(* Logix 5000 AddOnInstructionDefinition export Banner_QCM50_Param_v4; software revision 33.00 *)

TYPE Banner_IOL_Port_v4 :   // UDT that has all of the data items necessary to communicate with a specific Port on a IO-Link Master
STRUCT
   Port_Controlled : INT;   // Each bit represents a port on an IO-Link Master. Set to 1 to tell AOI to control that port.
   Port_Activate : INT;   // Each bit represents a port on an IO-Link Master. When ON that port will process any commands in queue.
   Port_Read : INT;   // Each bit represents a port on an IO-Link Master. Used to determine when device AOI has requested a Read command.
   Port_Write : INT;   // Each bit represents a port on an IO-Link Master. Used to determine when device AOI has requested a Write command.
   Port_RW_Complete : INT;   // Each bit represents a port on an IO-Link Master. Tells device AOI that Read or Write request has been completed.
   Port_Device_Read : INT;
   Data_Transfer : SINT[190];   // Array to transfer data from IO-Master to device AOIs.
END_STRUCT
END_TYPE

TYPE Banner_QCM50_Color_Tol_v4 :   // Color Tolerances for a QCM50.
STRUCT
   Ratio_Red : INT;   // 0 to 4095 = 0 to 100%
   Ratio_Green : INT;   // 0 to 4095 = 0 to 100%
   Energy : INT;   // 0 to 4095 = 0 to 100%
   Red_Tolerance : INT;   // 0 to 4095 = 0 to 100%
   Green_Tolerance : INT;   // 0 to 4095 = 0 to 100%
   Energy_Tolerance : INT;   // 0 to 4095 = 0 to 100%
END_STRUCT
END_TYPE

TYPE Banner_QCM50_Color_v4 :
STRUCT
   Tolerance : INT;   // 0 = Finest, 1 = 2nd level, 2 = 3rd level, 3 = 4th level, 4 = 5th level, 5 = 6th level, 6 = 7th level, 7 = 8th level, 8 = Roughest level
   NO_NC : SINT;   // 0 = NO, 1 = NC
   Function_Switching_Output : SINT;   // 0 = Disable, 1 = Output
   Energy_Evalution : SINT;   // 0 = Off, 1 = On
   Counter : DINT;   // 0 to 65535
   On_Delay : DINT;   // 0 to 65535
   Off_Delay : DINT;   // 0 to 65535
   Impulse_1Shot : DINT;   // 0 to 65535
   Connect_Colors : SINT;   // See IODD for more information.
END_STRUCT
END_TYPE

TYPE Banner_QCM50_RD_v4 :   // UDT that stores the Write Data for a QCM50.
STRUCT
   Master_Cycle_Time : INT;
   Min_Cycle_Time : INT;
   M_Sequence_Capability : INT;
   IO_Link_Version_ID : INT;
   Process_Data_Input_Length : INT;
   Process_Data_Output_Length : INT;
   Combined_Vendor_ID : DINT;   // IO-Link Vendor ID
   Vendor_ID1 : INT;
   Vendor_ID2 : INT;
   Combined_Device_ID : DINT;   // IO-Link Device ID
   Device_ID1 : INT;
   Device_ID2 : INT;
   Device_ID3 : INT;
   Serial_Number : STRING;
   Operating_Temp : INT;
   Max_Temp_Since_Restart : INT;
   Min_Temp_Since_Restart : INT;
   Max_Temp_Lifetime : INT;
   Min_Temp_Lifetime : INT;
   Operating_Hours : DINT;
   Counter_Switch_Cycle : DINT;
   Teach_Status : SINT;   // 0 = Idle, 1 to 3 = Success, 4 = Wait for Command, 5 = Busy, 7 = Error
   SP1_TP1 : SINT;   // 0 = -, 1 = Teach Successful.
   SP1_TP2 : SINT;   // 0 = -, 1 = Teach Successful.
   SP2_TP1 : SINT;   // 0 = -, 1 = Teach Successful.
   SP2_TP2 : SINT;   // 0 = -, 1 = Teach Successful.
   Current_Signal_Quality : INT;   // 0 to 100
END_STRUCT
END_TYPE

TYPE Banner_QCM50_v4 :   // All of the parameters for a QCM50.
STRUCT
   Initial_Global_Read : BOOL;   // Determines if all of the IO-Link data has been read into the PLC yet
   Command : INT;   // Value placed in here will activate a read or write to a specifc IO-Link Index
   Read_Data : Banner_QCM50_RD_v4;   // Read Only Data
   Write_Data : Banner_QCM50_WD_v4;   // Write Data
   Archive : Banner_QCM50_WD_v4;   // Archive of Write Data. Used to determine when data needs to be updated in the IO-Link Master.
   Reset : BOOL;   // Resets AOI. This will force a complete parameter read of the sensor.
END_STRUCT
END_TYPE

TYPE Banner_QCM50_WD_v4 :   // UDT that stores the Write Data for a Q4X.
STRUCT
   System_Command : INT;   // See IODD file for list of commands that can be activated via the System Command interface
   Parameter_Access_Lock : SINT;   // Write access to all parameters is prohibited while value is 1. Only this parameter can be adjusted when value is 1.
   Data_Storage_Lock : SINT;   // Automatic data storage is disabled when this value is equal to 1. Read access is not affected.
   Local_Parameterization_Lock : SINT;   // Parameterization via local control elements on device is disabled.
   Local_User_Interface_Lock : SINT;   // Operation of local user interface is disabled.
   Color_Setpoint : Banner_QCM50_Color_v4[13];
   Color1_Tolerances : Banner_QCM50_Color_Tol_v4[13];
   PNP_NPN : SINT;   // 0 = NPN, 1 = PNP, 2 = Auto
   Switching_Freq_Averaging : SINT;   // 0 = 3 Hz, 1 = 30 Hz, 2 = 100 Hz, 3 = 300 Hz, 4 = 500 Hz, 5 = 1500 Hz, 6 = 3000 Hz
   Binary_Output : SINT;   // 0 = Disable, 1 = Enable. NA for K1.
   Detection_Mode : SINT;   // 0 = Color Mode, 1 = Best Fit. NA for K1.
   Signal_Quality_Level : SINT;   // 10 to 90
   Process_Data_Mapping : SINT;   // 0 = Switching Channel, 1 = Color Values. NA for K1.
   Teach_Channel : SINT;   // Check IODD files for options. NA for K1.
   Input_Config : SINT;   // 0 = Disable Input, 2 = Key Lock, 3 = Trigger, 4 = External Teach. NA for K2 and K3.
   Screensaver : SINT;   // 0 = Screensaver Off, 1 = Screensaver On
   Rotate_Display : SINT;   // 0 = Display read from back, 1 = Dispalay read from front
END_STRUCT
END_TYPE

ADD_ON_INSTRUCTION Banner_QCM50_Param_v4   (* revision 4.0, vendor Banner Engineering *)
// AOI to read and write parameter data to an IO-Link QCM50.
VAR_IN_OUT
   QCM50 : Banner_QCM50_v4; {required}
   Port_Data : Banner_IOL_Port_v4; {required}
END_VAR
VAR_INPUT
   Port : INT; {required}   // Enter the Port number that this AOI is to work with.
   K : SINT; {required}   // 1,3,or 5. Based off number after the K in part number.
END_VAR
VAR
   Local_Control : DINT; {access None}
   Global_Read_Command_Value : INT; {access None}
   Global_Write_Command_Value : INT; {access None}
   Command_Being_Processed : BOOL; {access None}
   Update_Archive : BOOL; {access None}
   Index_Write_Inprocess : DINT; {access None}
   Index_Write_Control : DINT; {access None}
   Inprocess_Index : DINT; {access None}
   CR_Index : SINT; {access None}
   CWC3_Index : SINT; {access None}
   CWC2_Index : SINT; {access None}
   CWC1_Index : SINT; {access None}
   C_Limit : SINT[2]; {access None}
   ColorChange : SINT[3] := ([0] := 1, [1] := 7, [2] := 12); {access None}
   CW_Index : SINT; {access None}
END_VAR

ROUTINE Logic   (* ladder *)
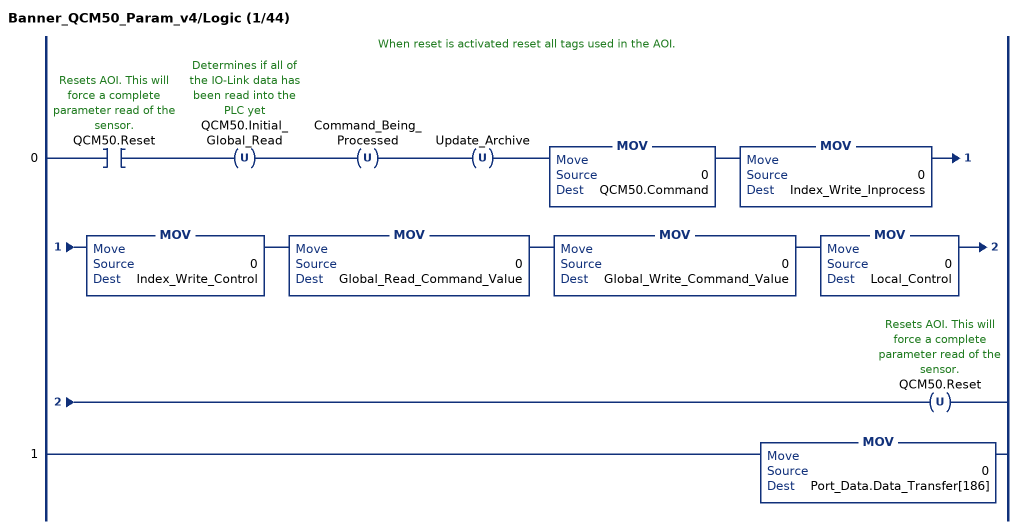
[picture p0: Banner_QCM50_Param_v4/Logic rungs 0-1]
   // When reset is activated reset all tags used in the AOI.
   0: XIC(QCM50.Reset)OTU(QCM50.Initial_Global_Read)OTU(Command_Being_Processed)OTU(Update_Archive)MOV(0,QCM50.Command)MOV(0,Index_Write_Inprocess)MOV(0,Index_Write_Control)MOV(0,Global_Read_Command_Value)MOV(0,Global_Write_Command_Value)MOV(0,Local_Control)OTU(QCM50.Reset);
   1: MOV(0,Port_Data.Data_Transfer[186]);
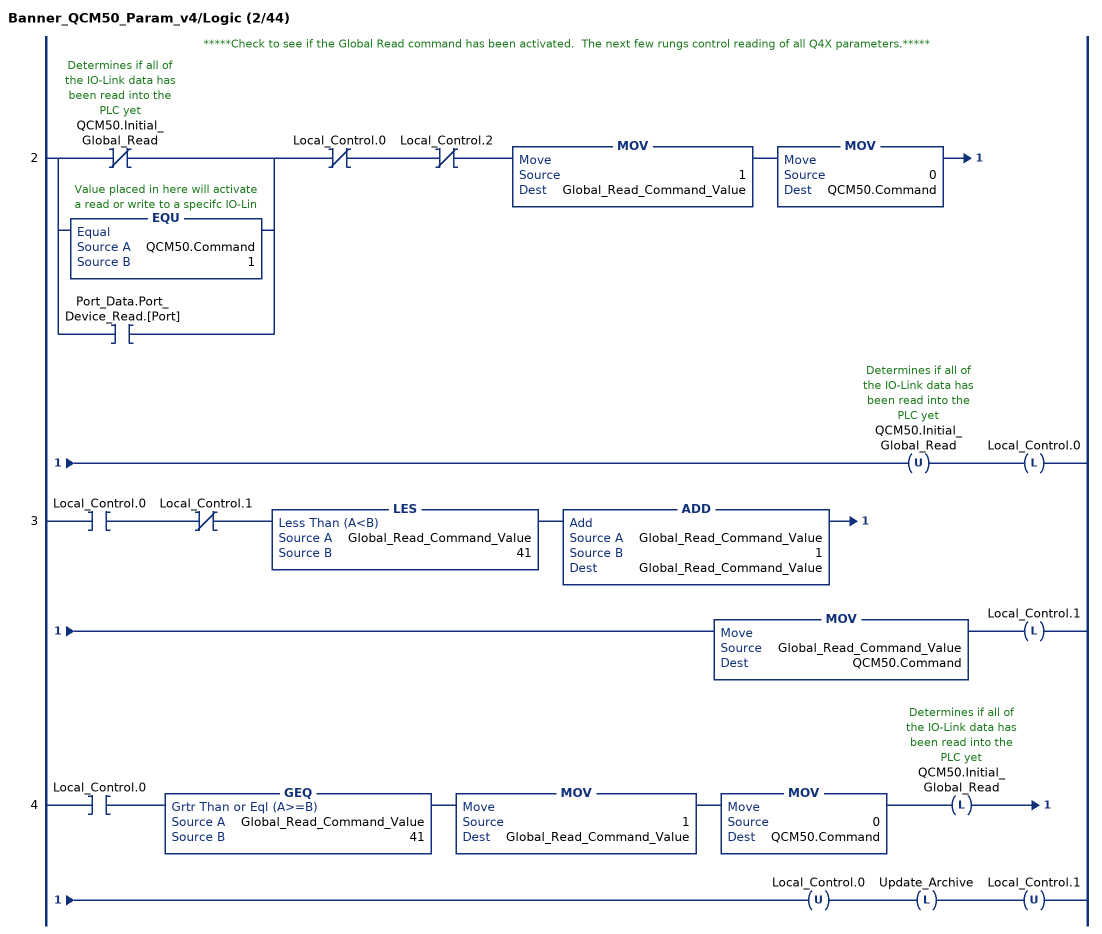
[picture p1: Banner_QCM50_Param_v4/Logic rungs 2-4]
   // *****Check to see if the Global Read command has been activated.  The next few rungs control reading of all Q4X parameters.*****
   2: [XIO(QCM50.Initial_Global_Read) ,EQU(QCM50.Command,1) ,XIC(Port_Data.Port_Device_Read.[Port]) ]XIO(Local_Control.0)XIO(Local_Control.2)MOV(1,Global_Read_Command_Value)MOV(0,QCM50.Command)OTU(QCM50.Initial_Global_Read)OTL(Local_Control.0);
   3: XIC(Local_Control.0)XIO(Local_Control.1)LES(Global_Read_Command_Value,41)ADD(Global_Read_Command_Value,1,Global_Read_Command_Value)MOV(Global_Read_Command_Value,QCM50.Command)OTL(Local_Control.1);
   4: XIC(Local_Control.0)GEQ(Global_Read_Command_Value,41)MOV(1,Global_Read_Command_Value)MOV(0,QCM50.Command)OTL(QCM50.Initial_Global_Read)OTU(Local_Control.0)OTL(Update_Archive)OTU(Local_Control.1);
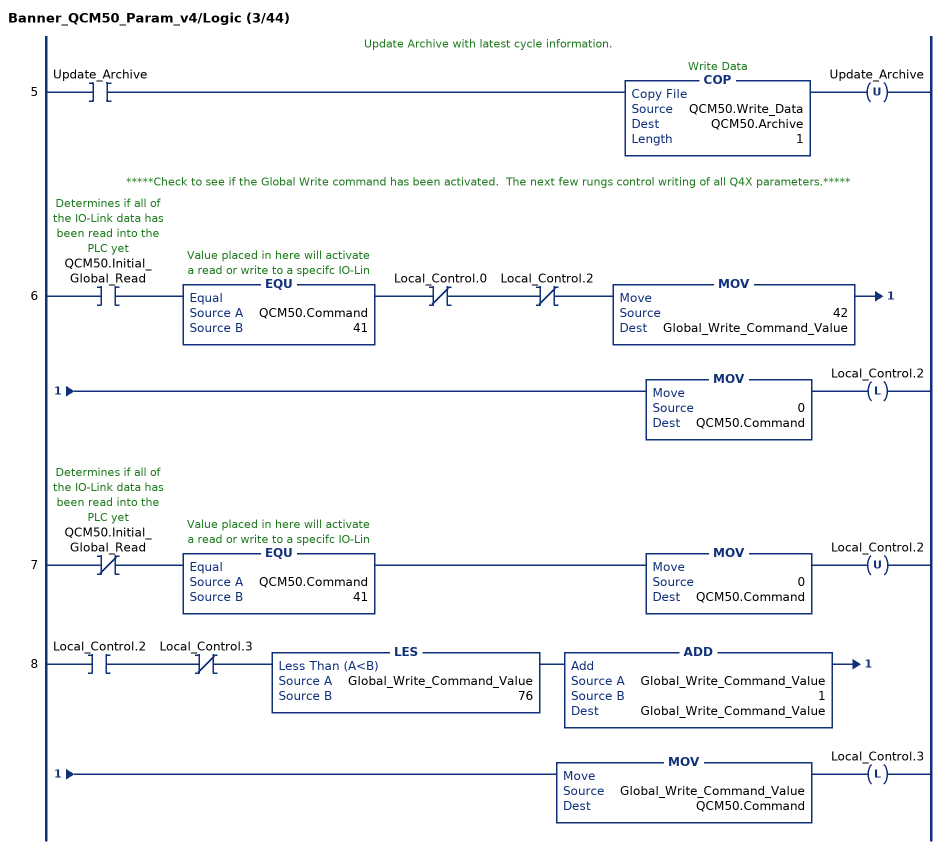
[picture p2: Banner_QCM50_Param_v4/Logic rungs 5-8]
   // Update Archive with latest cycle information.
   5: XIC(Update_Archive)COP(QCM50.Write_Data,QCM50.Archive,1)OTU(Update_Archive);
   // *****Check to see if the Global Write command has been activated.  The next few rungs control writing of all Q4X parameters.*****
   6: XIC(QCM50.Initial_Global_Read)EQU(QCM50.Command,41)XIO(Local_Control.0)XIO(Local_Control.2)MOV(42,Global_Write_Command_Value)MOV(0,QCM50.Command)OTL(Local_Control.2);
   7: XIO(QCM50.Initial_Global_Read)EQU(QCM50.Command,41)MOV(0,QCM50.Command)OTU(Local_Control.2);
   8: XIC(Local_Control.2)XIO(Local_Control.3)LES(Global_Write_Command_Value,76)ADD(Global_Write_Command_Value,1,Global_Write_Command_Value)MOV(Global_Write_Command_Value,QCM50.Command)OTL(Local_Control.3);
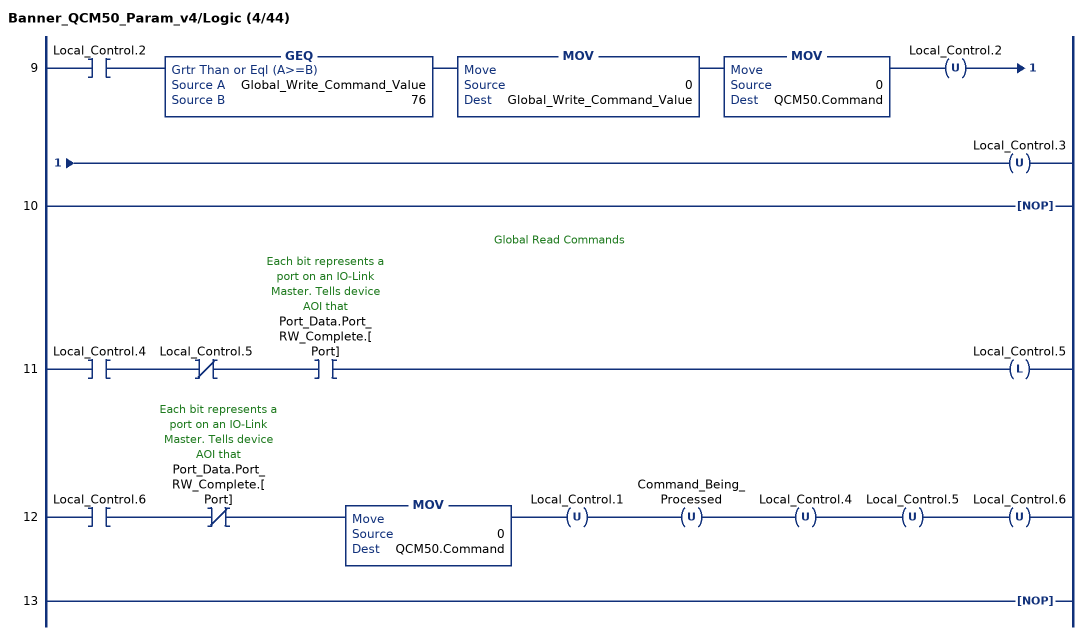
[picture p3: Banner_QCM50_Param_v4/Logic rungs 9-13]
   9: XIC(Local_Control.2)GEQ(Global_Write_Command_Value,76)MOV(0,Global_Write_Command_Value)MOV(0,QCM50.Command)OTU(Local_Control.2)OTU(Local_Control.3);
   10: NOP();
   // Global Read Commands
   11: XIC(Local_Control.4)XIO(Local_Control.5)XIC(Port_Data.Port_RW_Complete.[Port])OTL(Local_Control.5);
   12: XIC(Local_Control.6)XIO(Port_Data.Port_RW_Complete.[Port])MOV(0,QCM50.Command)OTU(Local_Control.1)OTU(Command_Being_Processed)OTU(Local_Control.4)OTU(Local_Control.5)OTU(Local_Control.6);
   13: NOP();
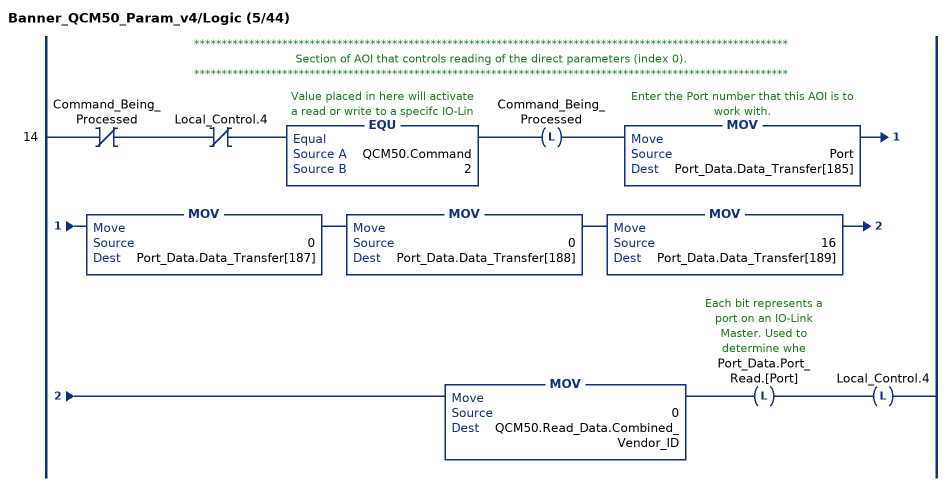
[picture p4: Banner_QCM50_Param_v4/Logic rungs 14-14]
   // ************************************************************************************************************
   // Section of AOI that controls reading of the direct parameters (index 0).
   // ************************************************************************************************************
   14: XIO(Command_Being_Processed)XIO(Local_Control.4)EQU(QCM50.Command,2)OTL(Command_Being_Processed)MOV(Port,Port_Data.Data_Transfer[185])MOV(0,Port_Data.Data_Transfer[187])MOV(0,Port_Data.Data_Transfer[188])MOV(16,Port_Data.Data_Transfer[189])MOV(0,QCM50.Read_Data.Combined_Vendor_ID)OTL(Port_Data.Port_Read.[Port])OTL(Local_Control.4);
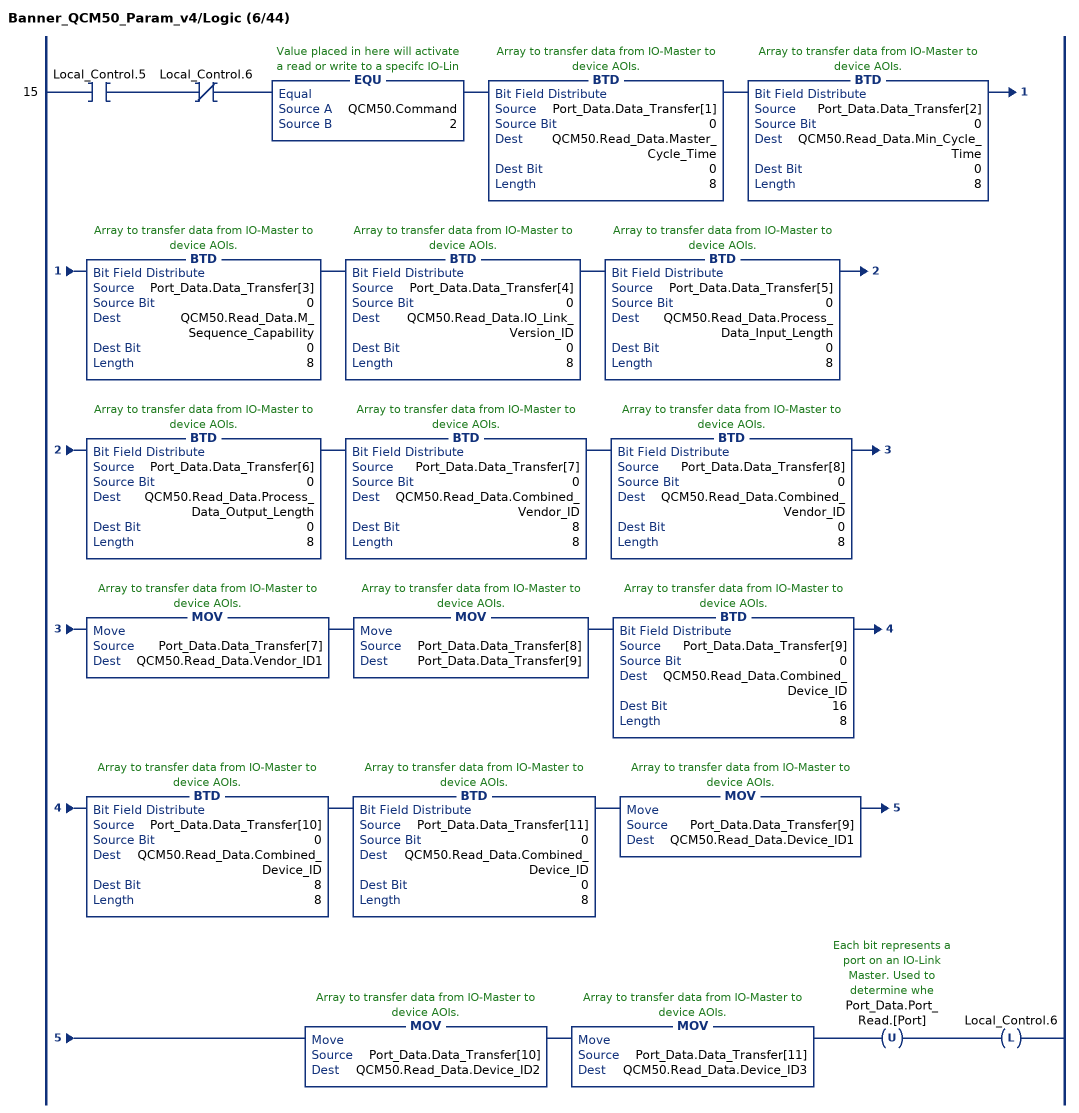
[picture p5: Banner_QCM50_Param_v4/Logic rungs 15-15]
   15: XIC(Local_Control.5)XIO(Local_Control.6)EQU(QCM50.Command,2)BTD(Port_Data.Data_Transfer[1],0,QCM50.Read_Data.Master_Cycle_Time,0,8)BTD(Port_Data.Data_Transfer[2],0,QCM50.Read_Data.Min_Cycle_Time,0,8)BTD(Port_Data.Data_Transfer[3],0,QCM50.Read_Data.M_Sequence_Capability,0,8)BTD(Port_Data.Data_Transfer[4],0,QCM50.Read_Data.IO_Link_Version_ID,0,8)BTD(Port_Data.Data_Transfer[5],0,QCM50.Read_Data.Process_Data_Input_Length,0,8)BTD(Port_Data.Data_Transfer[6],0,QCM50.Read_Data.Process_Data_Output_Length,0,8)BTD(Port_Data.Data_Transfer[7],0,QCM50.Read_Data.Combined_Vendor_ID,8,8)BTD(Port_Data.Data_Transfer[8],0,QCM50.Read_Data.Combined_Vendor_ID,0,8)MOV(Port_Data.Data_Transfer[7],QCM50.Read_Data.Vendor_ID1)MOV(Port_Data.Data_Transfer[8],Port_Data.Data_Transfer[9])BTD(Port_Data.Data_Transfer[9],0,QCM50.Read_Data.Combined_Device_ID,16,8)BTD(Port_Data.Data_Transfer[10],0,QCM50.Read_Data.Combined_Device_ID,8,8)BTD(Port_Data.Data_Transfer[11],0,QCM50.Read_Data.Combined_Device_ID,0,8)MOV(Port_Data.Data_Transfer[9],QCM50.Read_Data.Device_ID1)MOV(Port_Data.Data_Transfer[10],QCM50.Read_Data.Device_ID2)MOV(Port_Data.Data_Transfer[11],QCM50.Read_Data.Device_ID3)OTU(Port_Data.Port_Read.[Port])OTL(Local_Control.6);
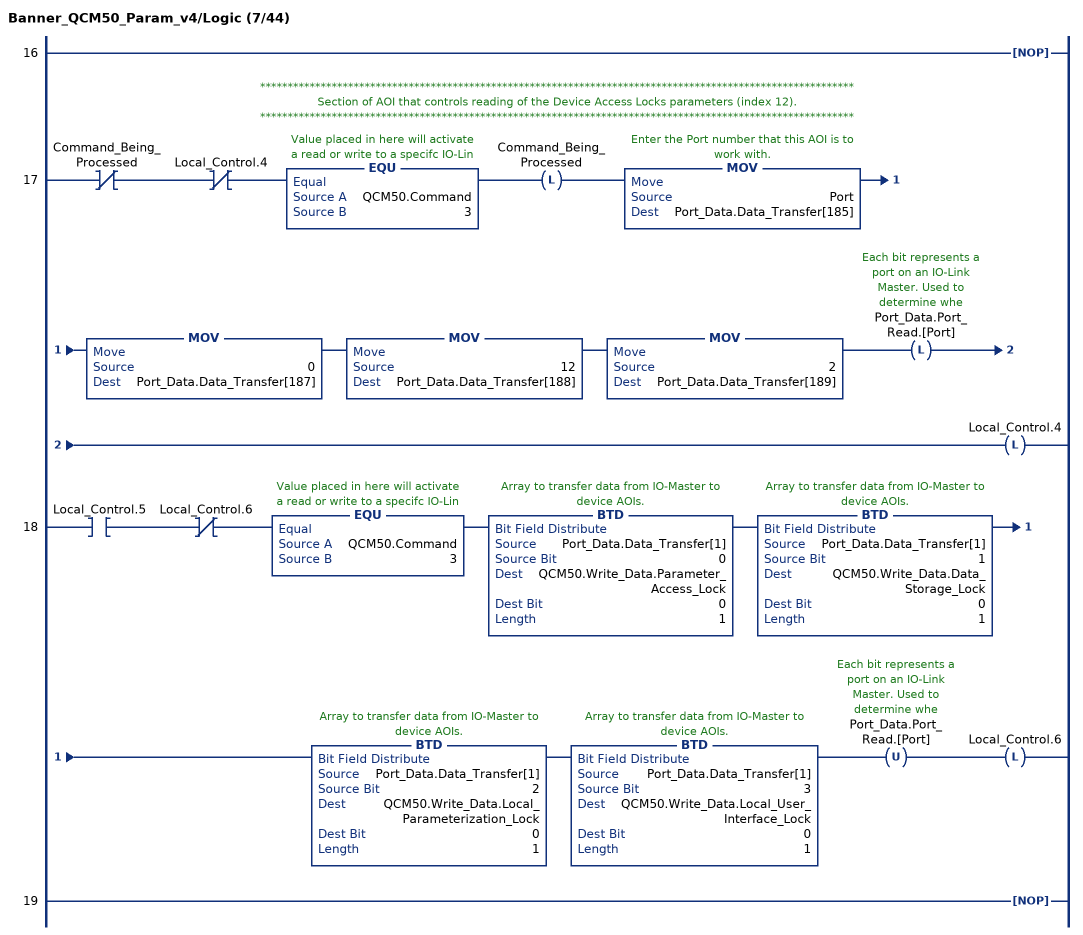
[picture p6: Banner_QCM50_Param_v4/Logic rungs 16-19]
   16: NOP();
   // ************************************************************************************************************
   // Section of AOI that controls reading of the Device Access Locks parameters (index 12).
   // ************************************************************************************************************
   17: XIO(Command_Being_Processed)XIO(Local_Control.4)EQU(QCM50.Command,3)OTL(Command_Being_Processed)MOV(Port,Port_Data.Data_Transfer[185])MOV(0,Port_Data.Data_Transfer[187])MOV(12,Port_Data.Data_Transfer[188])MOV(2,Port_Data.Data_Transfer[189])OTL(Port_Data.Port_Read.[Port])OTL(Local_Control.4);
   18: XIC(Local_Control.5)XIO(Local_Control.6)EQU(QCM50.Command,3)BTD(Port_Data.Data_Transfer[1],0,QCM50.Write_Data.Parameter_Access_Lock,0,1)BTD(Port_Data.Data_Transfer[1],1,QCM50.Write_Data.Data_Storage_Lock,0,1)BTD(Port_Data.Data_Transfer[1],2,QCM50.Write_Data.Local_Parameterization_Lock,0,1)BTD(Port_Data.Data_Transfer[1],3,QCM50.Write_Data.Local_User_Interface_Lock,0,1)OTU(Port_Data.Port_Read.[Port])OTL(Local_Control.6);
   19: NOP();
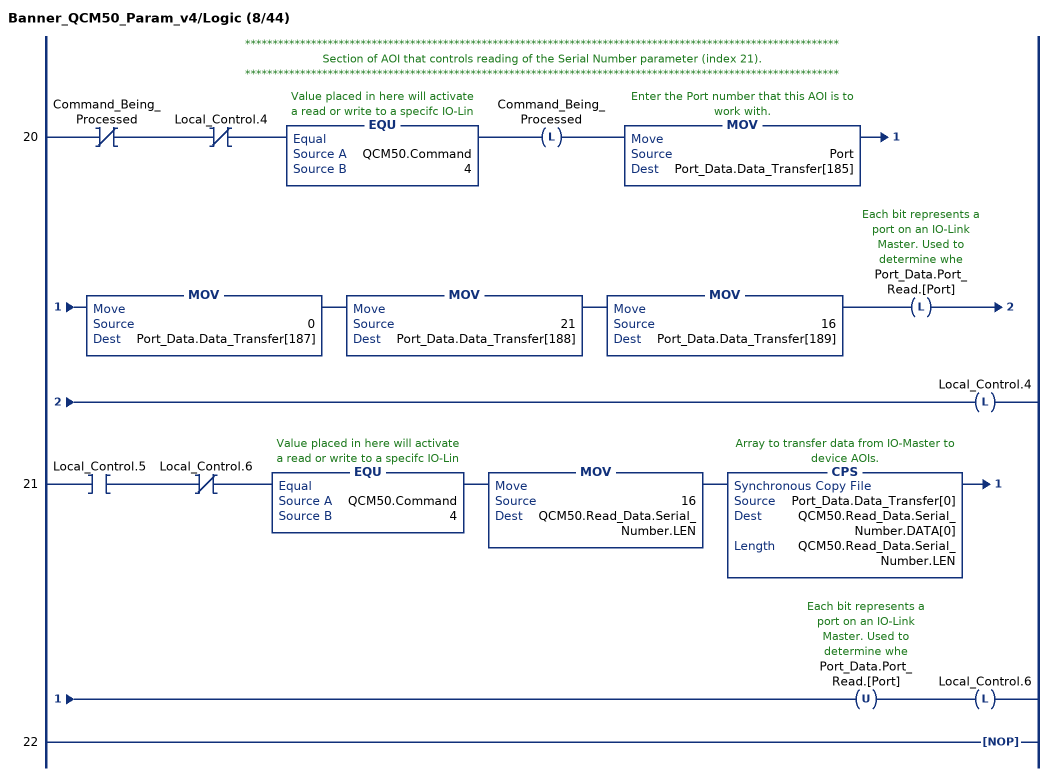
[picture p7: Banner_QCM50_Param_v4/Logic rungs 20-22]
   // ************************************************************************************************************
   // Section of AOI that controls reading of the Serial Number parameter (index 21).
   // ************************************************************************************************************
   20: XIO(Command_Being_Processed)XIO(Local_Control.4)EQU(QCM50.Command,4)OTL(Command_Being_Processed)MOV(Port,Port_Data.Data_Transfer[185])MOV(0,Port_Data.Data_Transfer[187])MOV(21,Port_Data.Data_Transfer[188])MOV(16,Port_Data.Data_Transfer[189])OTL(Port_Data.Port_Read.[Port])OTL(Local_Control.4);
   21: XIC(Local_Control.5)XIO(Local_Control.6)EQU(QCM50.Command,4)MOV(16,QCM50.Read_Data.Serial_Number.LEN)CPS(Port_Data.Data_Transfer[0],QCM50.Read_Data.Serial_Number.DATA[0],QCM50.Read_Data.Serial_Number.LEN)OTU(Port_Data.Port_Read.[Port])OTL(Local_Control.6);
   22: NOP();
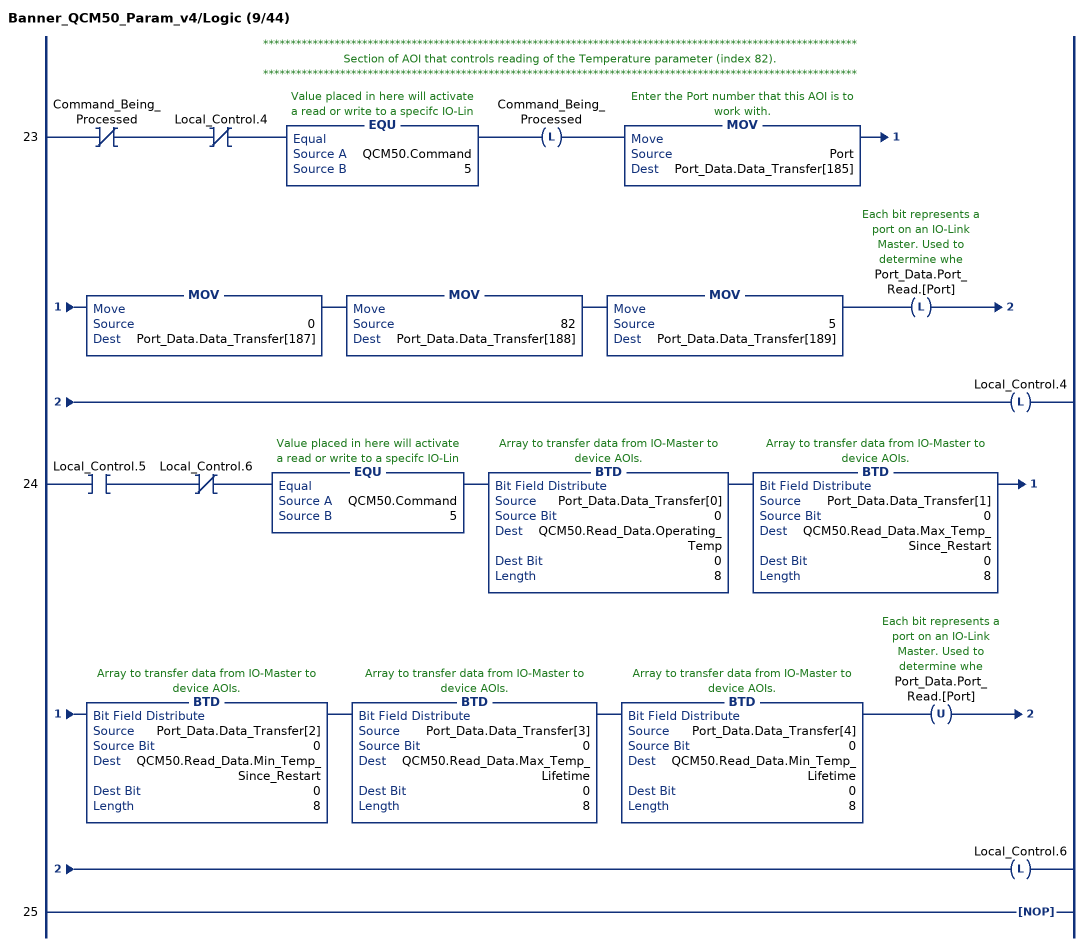
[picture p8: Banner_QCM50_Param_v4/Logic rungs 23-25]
   // ************************************************************************************************************
   // Section of AOI that controls reading of the Temperature parameter (index 82).
   // ************************************************************************************************************
   23: XIO(Command_Being_Processed)XIO(Local_Control.4)EQU(QCM50.Command,5)OTL(Command_Being_Processed)MOV(Port,Port_Data.Data_Transfer[185])MOV(0,Port_Data.Data_Transfer[187])MOV(82,Port_Data.Data_Transfer[188])MOV(5,Port_Data.Data_Transfer[189])OTL(Port_Data.Port_Read.[Port])OTL(Local_Control.4);
   24: XIC(Local_Control.5)XIO(Local_Control.6)EQU(QCM50.Command,5)BTD(Port_Data.Data_Transfer[0],0,QCM50.Read_Data.Operating_Temp,0,8)BTD(Port_Data.Data_Transfer[1],0,QCM50.Read_Data.Max_Temp_Since_Restart,0,8)BTD(Port_Data.Data_Transfer[2],0,QCM50.Read_Data.Min_Temp_Since_Restart,0,8)BTD(Port_Data.Data_Transfer[3],0,QCM50.Read_Data.Max_Temp_Lifetime,0,8)BTD(Port_Data.Data_Transfer[4],0,QCM50.Read_Data.Min_Temp_Lifetime,0,8)OTU(Port_Data.Port_Read.[Port])OTL(Local_Control.6);
   25: NOP();
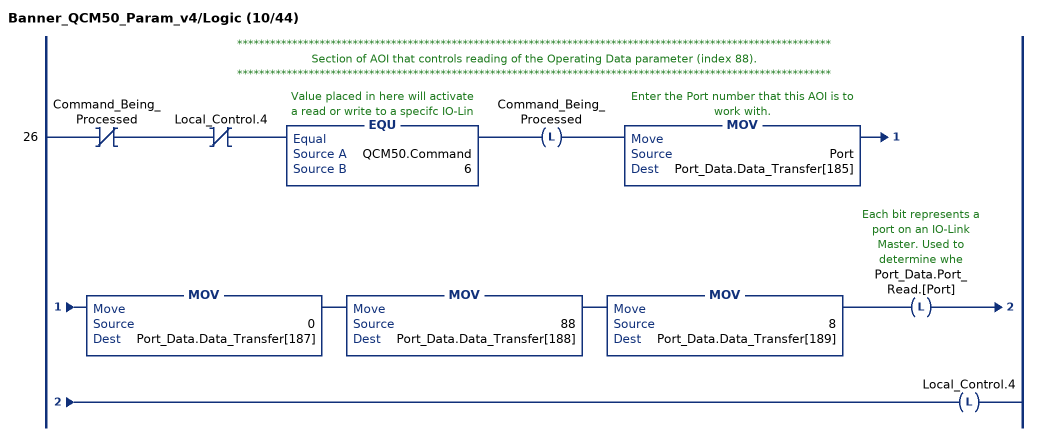
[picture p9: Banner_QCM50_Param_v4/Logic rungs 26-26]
   // ************************************************************************************************************
   // Section of AOI that controls reading of the Operating Data parameter (index 88).
   // ************************************************************************************************************
   26: XIO(Command_Being_Processed)XIO(Local_Control.4)EQU(QCM50.Command,6)OTL(Command_Being_Processed)MOV(Port,Port_Data.Data_Transfer[185])MOV(0,Port_Data.Data_Transfer[187])MOV(88,Port_Data.Data_Transfer[188])MOV(8,Port_Data.Data_Transfer[189])OTL(Port_Data.Port_Read.[Port])OTL(Local_Control.4);
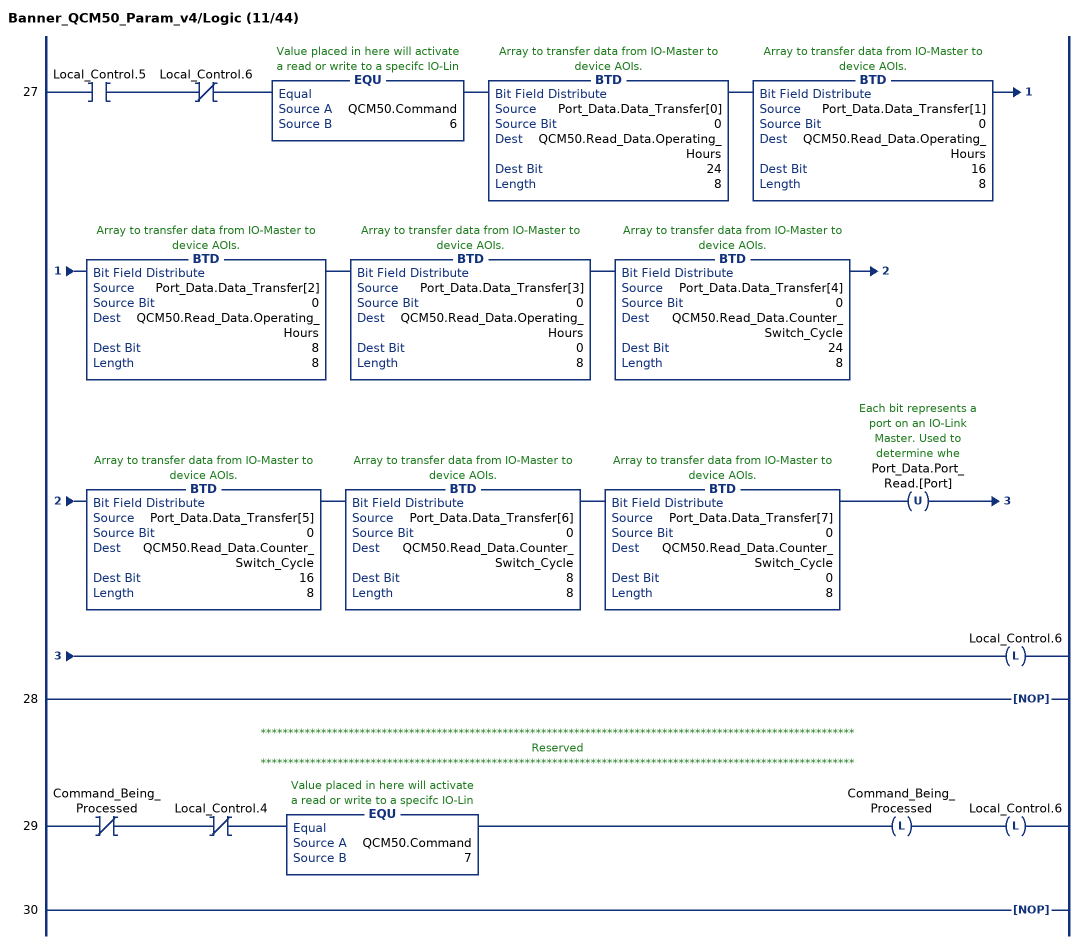
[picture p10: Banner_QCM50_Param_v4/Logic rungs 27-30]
   27: XIC(Local_Control.5)XIO(Local_Control.6)EQU(QCM50.Command,6)BTD(Port_Data.Data_Transfer[0],0,QCM50.Read_Data.Operating_Hours,24,8)BTD(Port_Data.Data_Transfer[1],0,QCM50.Read_Data.Operating_Hours,16,8)BTD(Port_Data.Data_Transfer[2],0,QCM50.Read_Data.Operating_Hours,8,8)BTD(Port_Data.Data_Transfer[3],0,QCM50.Read_Data.Operating_Hours,0,8)BTD(Port_Data.Data_Transfer[4],0,QCM50.Read_Data.Counter_Switch_Cycle,24,8)BTD(Port_Data.Data_Transfer[5],0,QCM50.Read_Data.Counter_Switch_Cycle,16,8)BTD(Port_Data.Data_Transfer[6],0,QCM50.Read_Data.Counter_Switch_Cycle,8,8)BTD(Port_Data.Data_Transfer[7],0,QCM50.Read_Data.Counter_Switch_Cycle,0,8)OTU(Port_Data.Port_Read.[Port])OTL(Local_Control.6);
   28: NOP();
   // ************************************************************************************************************
   // Reserved
   // ************************************************************************************************************
   29: XIO(Command_Being_Processed)XIO(Local_Control.4)EQU(QCM50.Command,7)OTL(Command_Being_Processed)OTL(Local_Control.6);
   30: NOP();
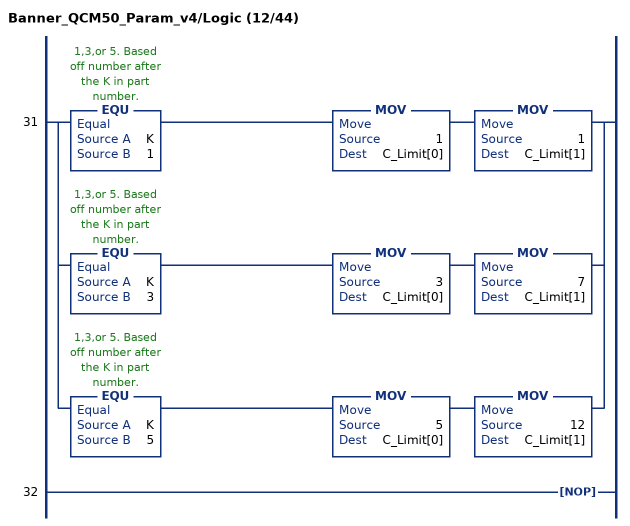
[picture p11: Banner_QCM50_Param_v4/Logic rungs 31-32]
   31: [EQU(K,1) MOV(1,C_Limit[0]) MOV(1,C_Limit[1]) ,EQU(K,3) MOV(3,C_Limit[0]) MOV(7,C_Limit[1]) ,EQU(K,5) MOV(5,C_Limit[0]) MOV(12,C_Limit[1]) ];
   32: NOP();
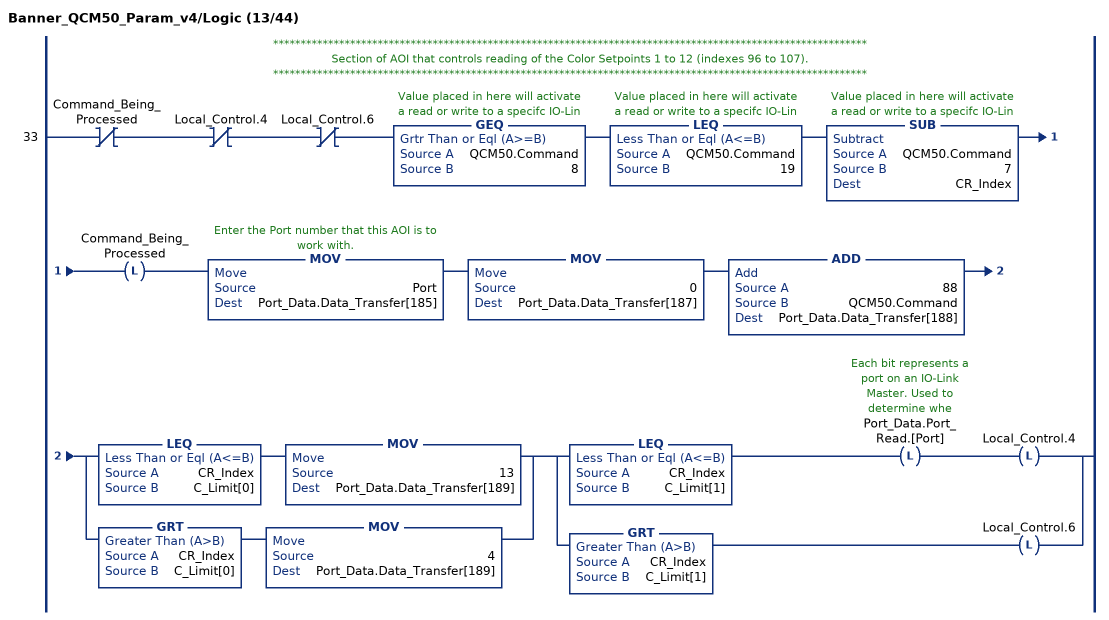
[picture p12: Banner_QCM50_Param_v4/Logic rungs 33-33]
   // ************************************************************************************************************
   // Section of AOI that controls reading of the Color Setpoints 1 to 12 (indexes 96 to 107).
   // ************************************************************************************************************
   33: XIO(Command_Being_Processed)XIO(Local_Control.4)XIO(Local_Control.6)GEQ(QCM50.Command,8)LEQ(QCM50.Command,19)SUB(QCM50.Command,7,CR_Index)OTL(Command_Being_Processed)MOV(Port,Port_Data.Data_Transfer[185])MOV(0,Port_Data.Data_Transfer[187])ADD(88,QCM50.Command,Port_Data.Data_Transfer[188])[LEQ(CR_Index,C_Limit[0]) MOV(13,Port_Data.Data_Transfer[189]) ,GRT(CR_Index,C_Limit[0]) MOV(4,Port_Data.Data_Transfer[189]) ][LEQ(CR_Index,C_Limit[1]) OTL(Port_Data.Port_Read.[Port]) OTL(Local_Control.4) ,GRT(CR_Index,C_Limit[1]) OTL(Local_Control.6) ];
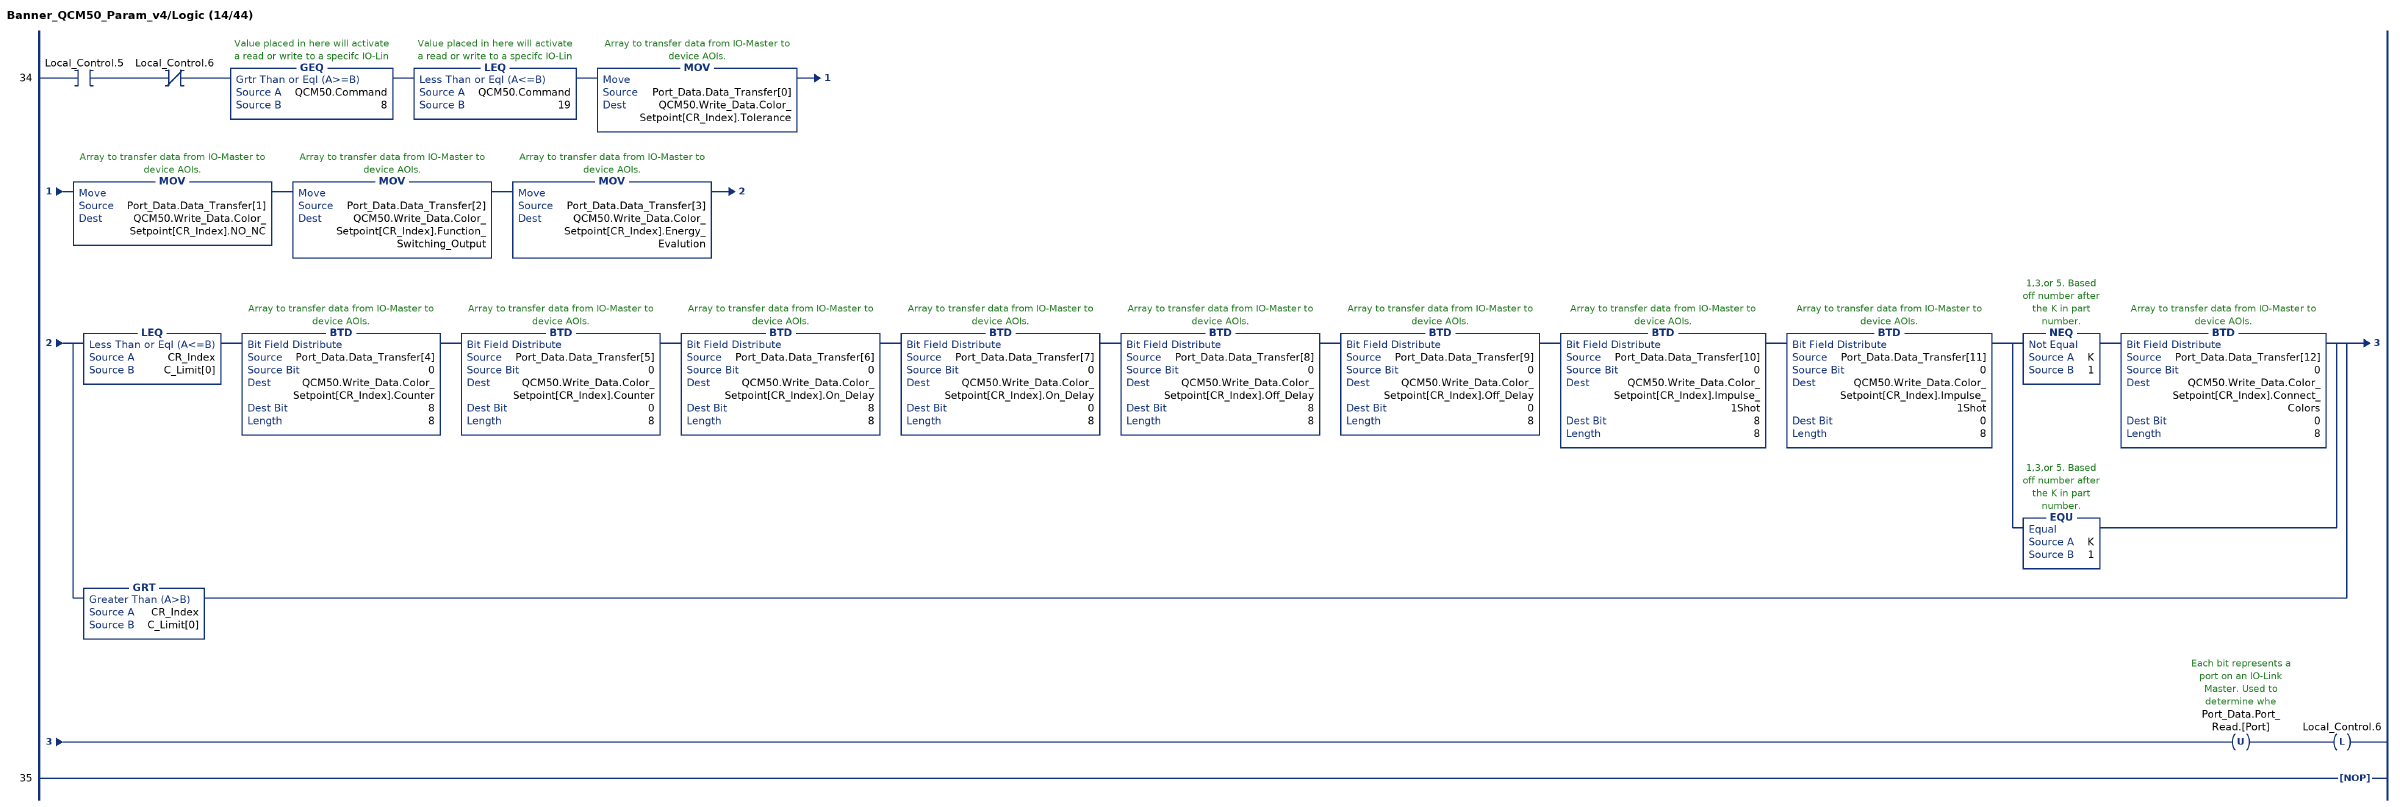
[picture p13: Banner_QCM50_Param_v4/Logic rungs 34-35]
   34: XIC(Local_Control.5)XIO(Local_Control.6)GEQ(QCM50.Command,8)LEQ(QCM50.Command,19)MOV(Port_Data.Data_Transfer[0],QCM50.Write_Data.Color_Setpoint[CR_Index].Tolerance)MOV(Port_Data.Data_Transfer[1],QCM50.Write_Data.Color_Setpoint[CR_Index].NO_NC)MOV(Port_Data.Data_Transfer[2],QCM50.Write_Data.Color_Setpoint[CR_Index].Function_Switching_Output)MOV(Port_Data.Data_Transfer[3],QCM50.Write_Data.Color_Setpoint[CR_Index].Energy_Evalution)[LEQ(CR_Index,C_Limit[0]) BTD(Port_Data.Data_Transfer[4],0,QCM50.Write_Data.Color_Setpoint[CR_Index].Counter,8,8) BTD(Port_Data.Data_Transfer[5],0,QCM50.Write_Data.Color_Setpoint[CR_Index].Counter,0,8) BTD(Port_Data.Data_Transfer[6],0,QCM50.Write_Data.Color_Setpoint[CR_Index].On_Delay,8,8) BTD(Port_Data.Data_Transfer[7],0,QCM50.Write_Data.Color_Setpoint[CR_Index].On_Delay,0,8) BTD(Port_Data.Data_Transfer[8],0,QCM50.Write_Data.Color_Setpoint[CR_Index].Off_Delay,8,8) BTD(Port_Data.Data_Transfer[9],0,QCM50.Write_Data.Color_Setpoint[CR_Index].Off_Delay,0,8) BTD(Port_Data.Data_Transfer[10],0,QCM50.Write_Data.Color_Setpoint[CR_Index].Impulse_1Shot,8,8) BTD(Port_Data.Data_Transfer[11],0,QCM50.Write_Data.Color_Setpoint[CR_Index].Impulse_1Shot,0,8) [NEQ(K,1) BTD(Port_Data.Data_Transfer[12],0,QCM50.Write_Data.Color_Setpoint[CR_Index].Connect_Colors,0,8) ,EQU(K,1) ] ,GRT(CR_Index,C_Limit[0]) ]OTU(Port_Data.Port_Read.[Port])OTL(Local_Control.6);
   35: NOP();
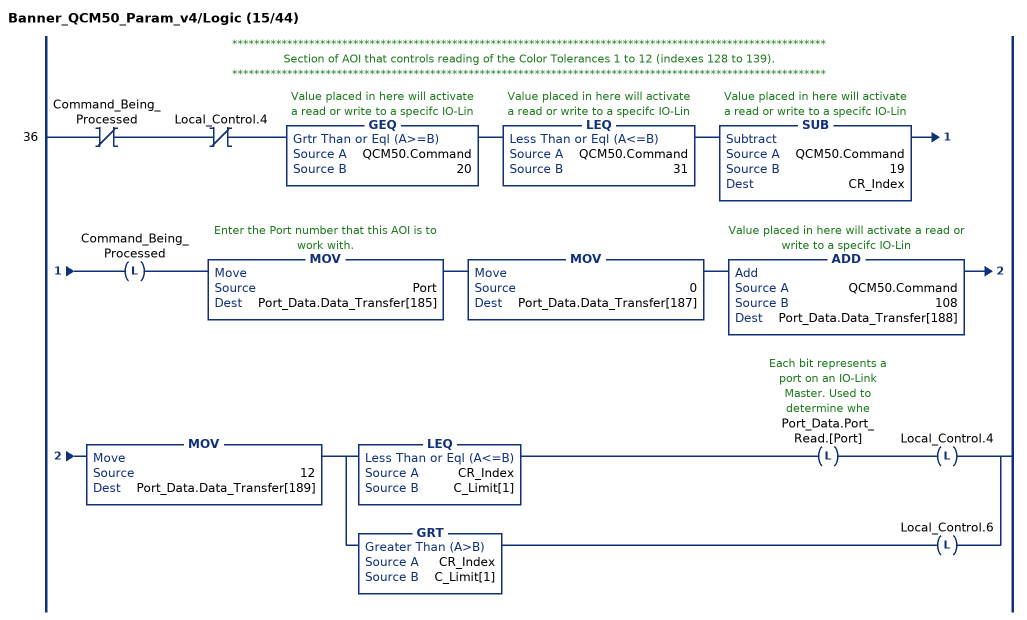
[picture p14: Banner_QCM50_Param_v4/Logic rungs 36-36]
   // ************************************************************************************************************
   // Section of AOI that controls reading of the Color Tolerances 1 to 12 (indexes 128 to 139).
   // ************************************************************************************************************
   36: XIO(Command_Being_Processed)XIO(Local_Control.4)GEQ(QCM50.Command,20)LEQ(QCM50.Command,31)SUB(QCM50.Command,19,CR_Index)OTL(Command_Being_Processed)MOV(Port,Port_Data.Data_Transfer[185])MOV(0,Port_Data.Data_Transfer[187])ADD(QCM50.Command,108,Port_Data.Data_Transfer[188])MOV(12,Port_Data.Data_Transfer[189])[LEQ(CR_Index,C_Limit[1]) OTL(Port_Data.Port_Read.[Port]) OTL(Local_Control.4) ,GRT(CR_Index,C_Limit[1]) OTL(Local_Control.6) ];
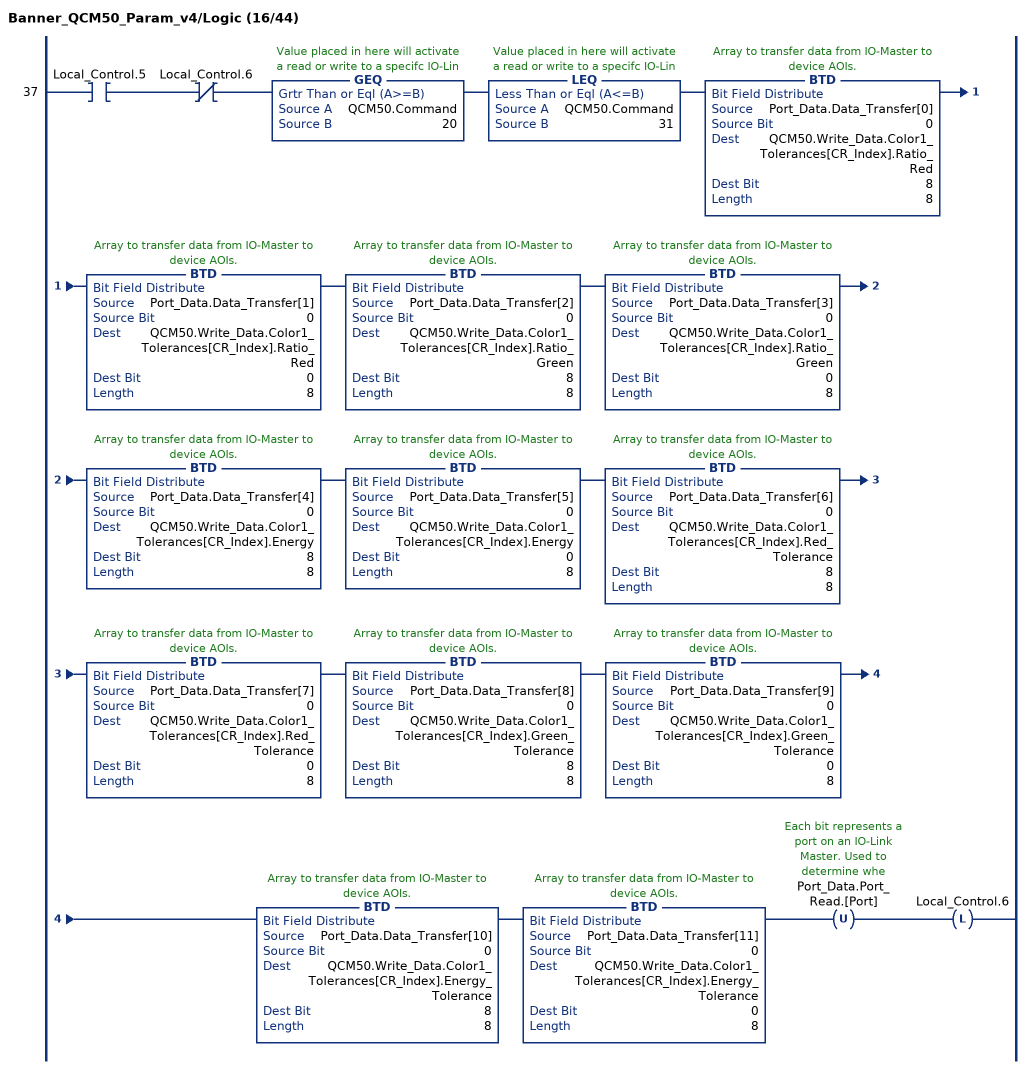
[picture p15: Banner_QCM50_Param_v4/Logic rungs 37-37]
   37: XIC(Local_Control.5)XIO(Local_Control.6)GEQ(QCM50.Command,20)LEQ(QCM50.Command,31)BTD(Port_Data.Data_Transfer[0],0,QCM50.Write_Data.Color1_Tolerances[CR_Index].Ratio_Red,8,8)BTD(Port_Data.Data_Transfer[1],0,QCM50.Write_Data.Color1_Tolerances[CR_Index].Ratio_Red,0,8)BTD(Port_Data.Data_Transfer[2],0,QCM50.Write_Data.Color1_Tolerances[CR_Index].Ratio_Green,8,8)BTD(Port_Data.Data_Transfer[3],0,QCM50.Write_Data.Color1_Tolerances[CR_Index].Ratio_Green,0,8)BTD(Port_Data.Data_Transfer[4],0,QCM50.Write_Data.Color1_Tolerances[CR_Index].Energy,8,8)BTD(Port_Data.Data_Transfer[5],0,QCM50.Write_Data.Color1_Tolerances[CR_Index].Energy,0,8)BTD(Port_Data.Data_Transfer[6],0,QCM50.Write_Data.Color1_Tolerances[CR_Index].Red_Tolerance,8,8)BTD(Port_Data.Data_Transfer[7],0,QCM50.Write_Data.Color1_Tolerances[CR_Index].Red_Tolerance,0,8)BTD(Port_Data.Data_Transfer[8],0,QCM50.Write_Data.Color1_Tolerances[CR_Index].Green_Tolerance,8,8)BTD(Port_Data.Data_Transfer[9],0,QCM50.Write_Data.Color1_Tolerances[CR_Index].Green_Tolerance,0,8)BTD(Port_Data.Data_Transfer[10],0,QCM50.Write_Data.Color1_Tolerances[CR_Index].Energy_Tolerance,8,8)BTD(Port_Data.Data_Transfer[11],0,QCM50.Write_Data.Color1_Tolerances[CR_Index].Energy_Tolerance,0,8)OTU(Port_Data.Port_Read.[Port])OTL(Local_Control.6);
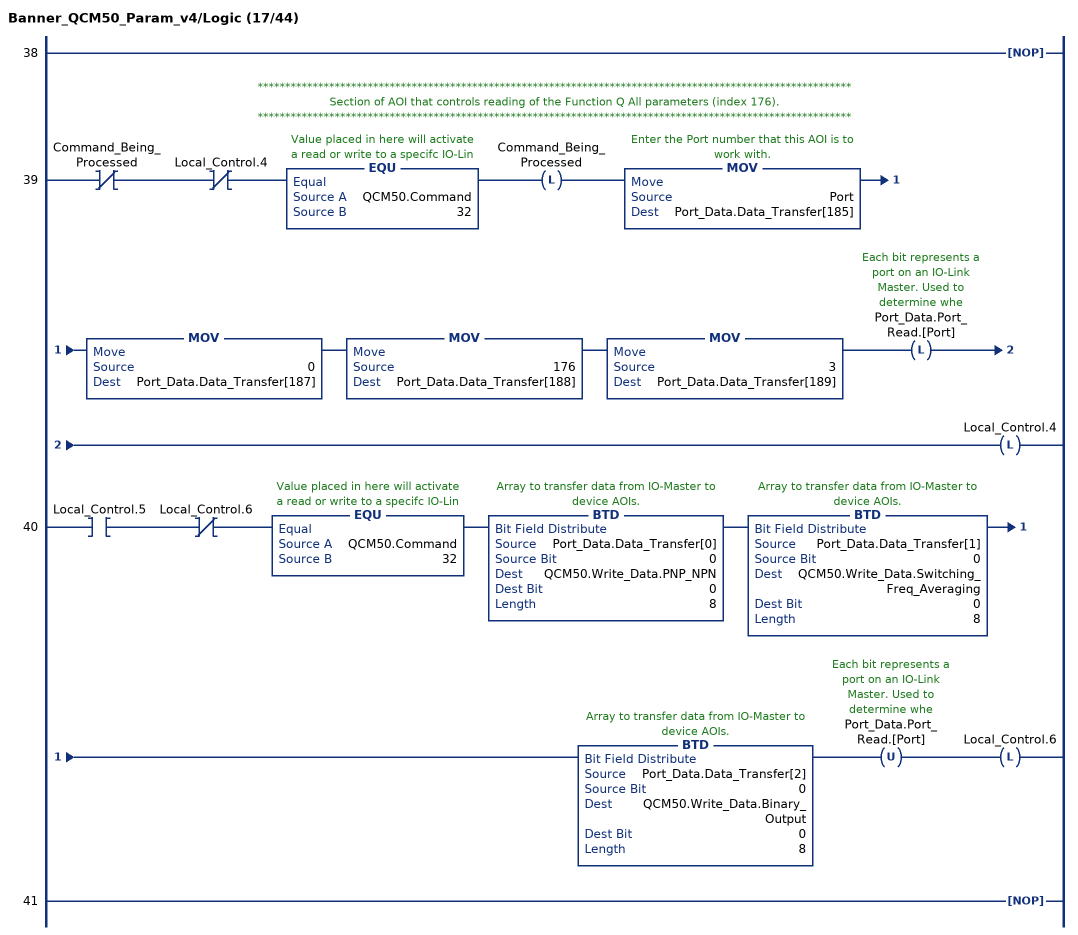
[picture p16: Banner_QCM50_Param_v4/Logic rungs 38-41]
   38: NOP();
   // ************************************************************************************************************
   // Section of AOI that controls reading of the Function Q All parameters (index 176).
   // ************************************************************************************************************
   39: XIO(Command_Being_Processed)XIO(Local_Control.4)EQU(QCM50.Command,32)OTL(Command_Being_Processed)MOV(Port,Port_Data.Data_Transfer[185])MOV(0,Port_Data.Data_Transfer[187])MOV(176,Port_Data.Data_Transfer[188])MOV(3,Port_Data.Data_Transfer[189])OTL(Port_Data.Port_Read.[Port])OTL(Local_Control.4);
   40: XIC(Local_Control.5)XIO(Local_Control.6)EQU(QCM50.Command,32)BTD(Port_Data.Data_Transfer[0],0,QCM50.Write_Data.PNP_NPN,0,8)BTD(Port_Data.Data_Transfer[1],0,QCM50.Write_Data.Switching_Freq_Averaging,0,8)BTD(Port_Data.Data_Transfer[2],0,QCM50.Write_Data.Binary_Output,0,8)OTU(Port_Data.Port_Read.[Port])OTL(Local_Control.6);
   41: NOP();
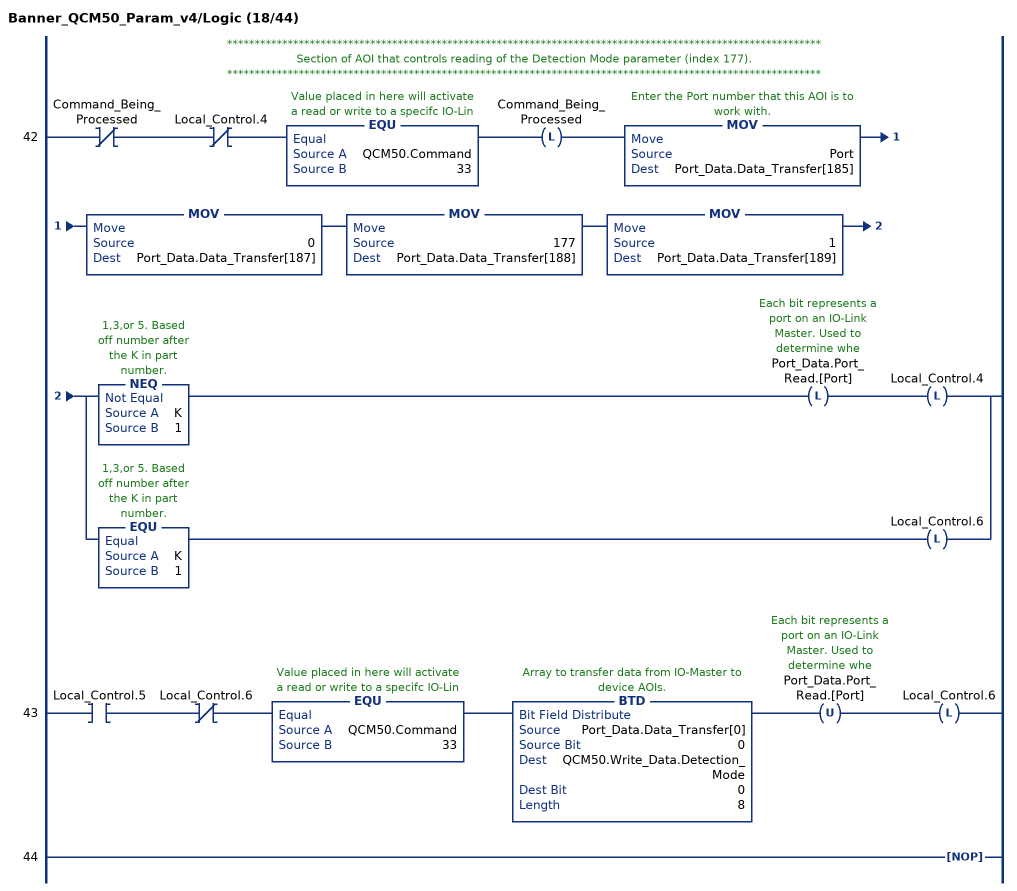
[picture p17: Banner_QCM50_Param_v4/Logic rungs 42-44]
   // ************************************************************************************************************
   // Section of AOI that controls reading of the Detection Mode parameter (index 177).
   // ************************************************************************************************************
   42: XIO(Command_Being_Processed)XIO(Local_Control.4)EQU(QCM50.Command,33)OTL(Command_Being_Processed)MOV(Port,Port_Data.Data_Transfer[185])MOV(0,Port_Data.Data_Transfer[187])MOV(177,Port_Data.Data_Transfer[188])MOV(1,Port_Data.Data_Transfer[189])[NEQ(K,1) OTL(Port_Data.Port_Read.[Port]) OTL(Local_Control.4) ,EQU(K,1) OTL(Local_Control.6) ];
   43: XIC(Local_Control.5)XIO(Local_Control.6)EQU(QCM50.Command,33)BTD(Port_Data.Data_Transfer[0],0,QCM50.Write_Data.Detection_Mode,0,8)OTU(Port_Data.Port_Read.[Port])OTL(Local_Control.6);
   44: NOP();
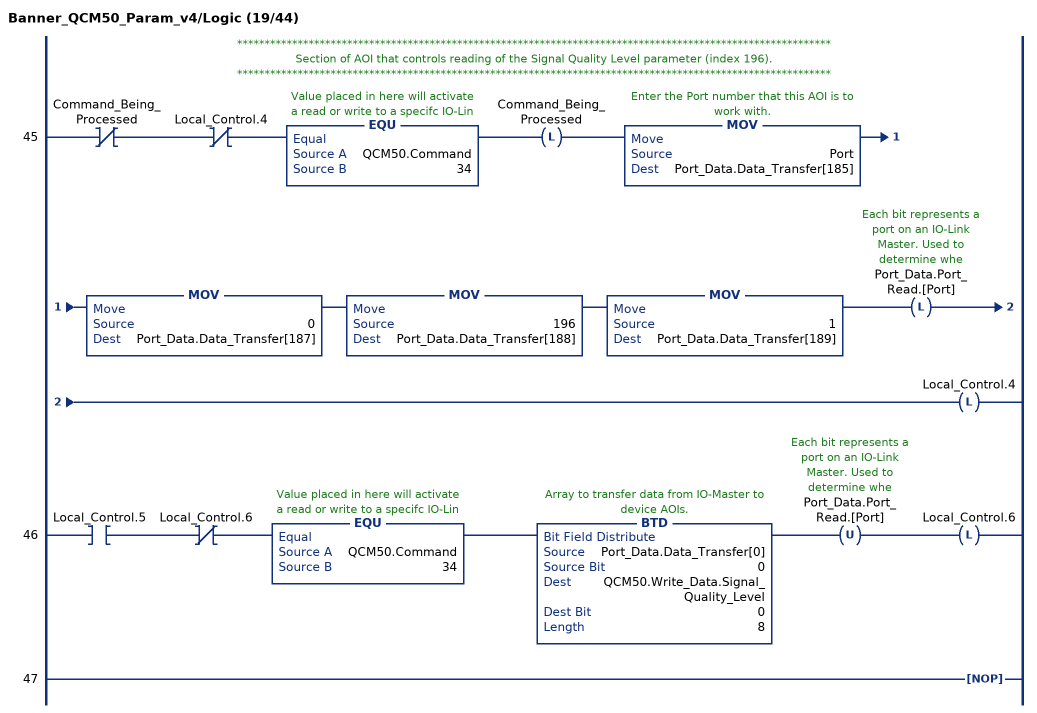
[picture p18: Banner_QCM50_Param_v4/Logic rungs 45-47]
   // ************************************************************************************************************
   // Section of AOI that controls reading of the Signal Quality Level parameter (index 196).
   // ************************************************************************************************************
   45: XIO(Command_Being_Processed)XIO(Local_Control.4)EQU(QCM50.Command,34)OTL(Command_Being_Processed)MOV(Port,Port_Data.Data_Transfer[185])MOV(0,Port_Data.Data_Transfer[187])MOV(196,Port_Data.Data_Transfer[188])MOV(1,Port_Data.Data_Transfer[189])OTL(Port_Data.Port_Read.[Port])OTL(Local_Control.4);
   46: XIC(Local_Control.5)XIO(Local_Control.6)EQU(QCM50.Command,34)BTD(Port_Data.Data_Transfer[0],0,QCM50.Write_Data.Signal_Quality_Level,0,8)OTU(Port_Data.Port_Read.[Port])OTL(Local_Control.6);
   47: NOP();
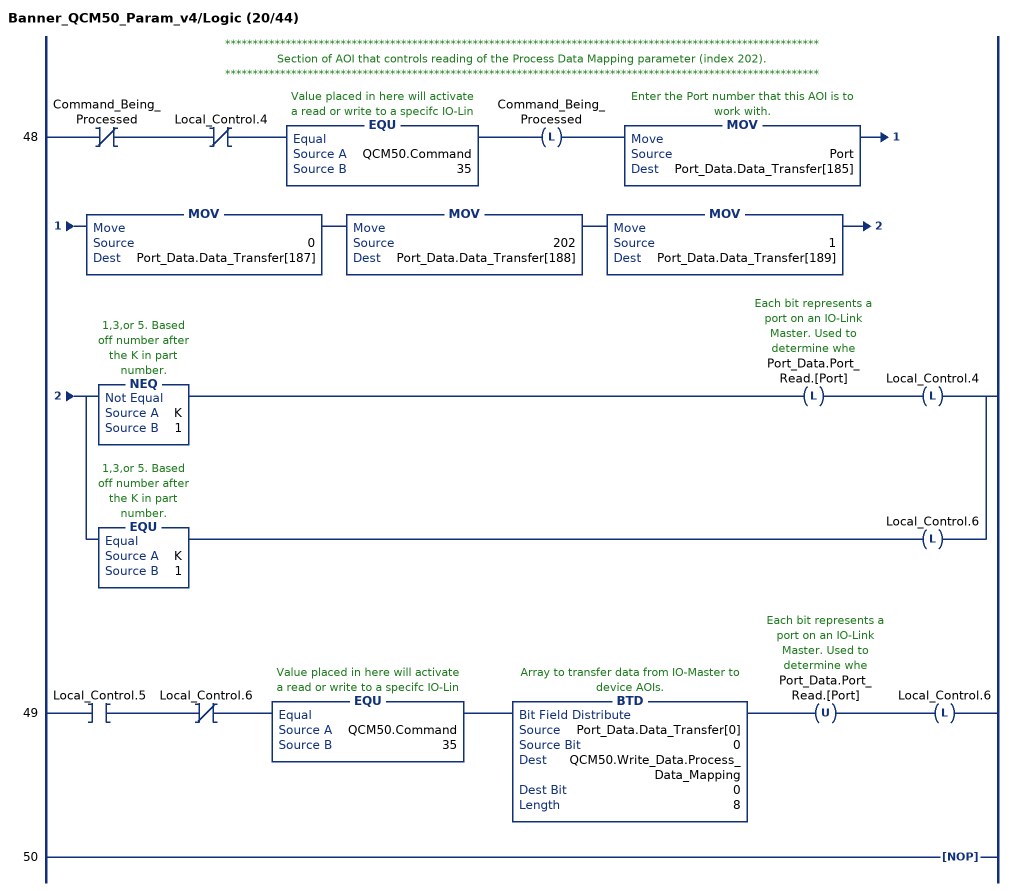
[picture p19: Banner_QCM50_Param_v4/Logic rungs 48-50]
   // ************************************************************************************************************
   // Section of AOI that controls reading of the Process Data Mapping parameter (index 202).
   // ************************************************************************************************************
   48: XIO(Command_Being_Processed)XIO(Local_Control.4)EQU(QCM50.Command,35)OTL(Command_Being_Processed)MOV(Port,Port_Data.Data_Transfer[185])MOV(0,Port_Data.Data_Transfer[187])MOV(202,Port_Data.Data_Transfer[188])MOV(1,Port_Data.Data_Transfer[189])[NEQ(K,1) OTL(Port_Data.Port_Read.[Port]) OTL(Local_Control.4) ,EQU(K,1) OTL(Local_Control.6) ];
   49: XIC(Local_Control.5)XIO(Local_Control.6)EQU(QCM50.Command,35)BTD(Port_Data.Data_Transfer[0],0,QCM50.Write_Data.Process_Data_Mapping,0,8)OTU(Port_Data.Port_Read.[Port])OTL(Local_Control.6);
   50: NOP();
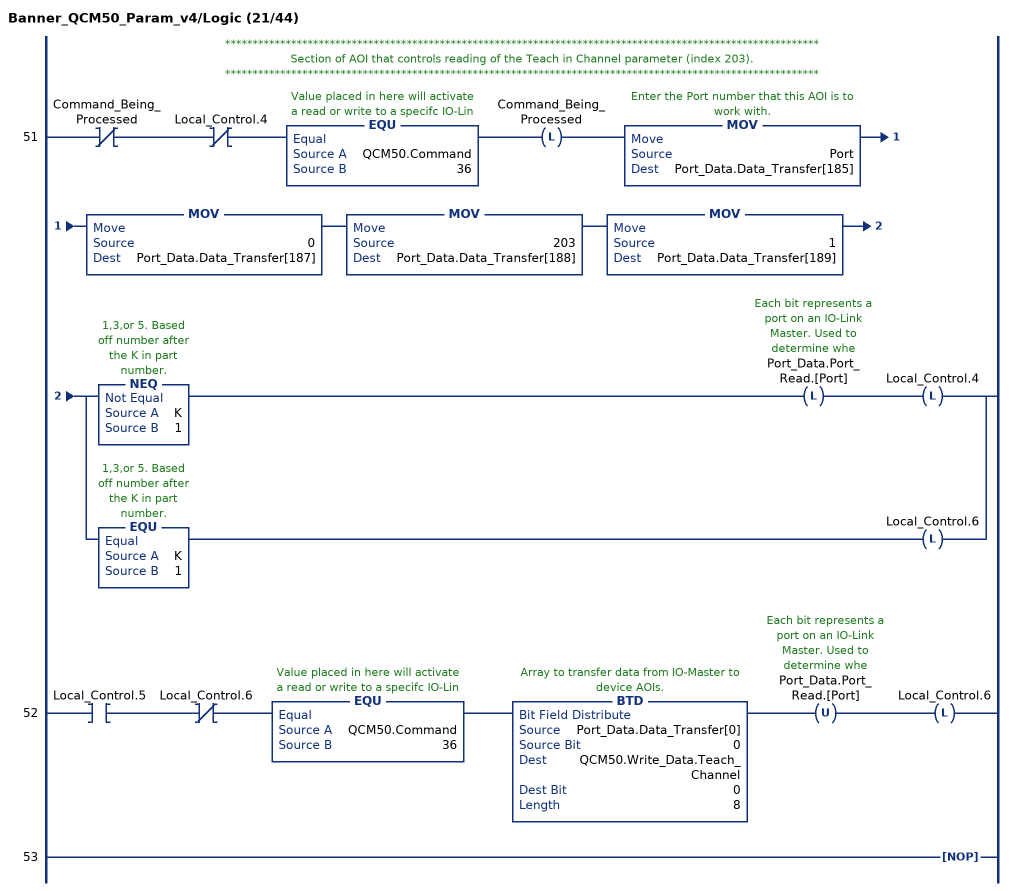
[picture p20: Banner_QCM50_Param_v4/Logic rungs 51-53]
   // ************************************************************************************************************
   // Section of AOI that controls reading of the Teach in Channel parameter (index 203).
   // ************************************************************************************************************
   51: XIO(Command_Being_Processed)XIO(Local_Control.4)EQU(QCM50.Command,36)OTL(Command_Being_Processed)MOV(Port,Port_Data.Data_Transfer[185])MOV(0,Port_Data.Data_Transfer[187])MOV(203,Port_Data.Data_Transfer[188])MOV(1,Port_Data.Data_Transfer[189])[NEQ(K,1) OTL(Port_Data.Port_Read.[Port]) OTL(Local_Control.4) ,EQU(K,1) OTL(Local_Control.6) ];
   52: XIC(Local_Control.5)XIO(Local_Control.6)EQU(QCM50.Command,36)BTD(Port_Data.Data_Transfer[0],0,QCM50.Write_Data.Teach_Channel,0,8)OTU(Port_Data.Port_Read.[Port])OTL(Local_Control.6);
   53: NOP();
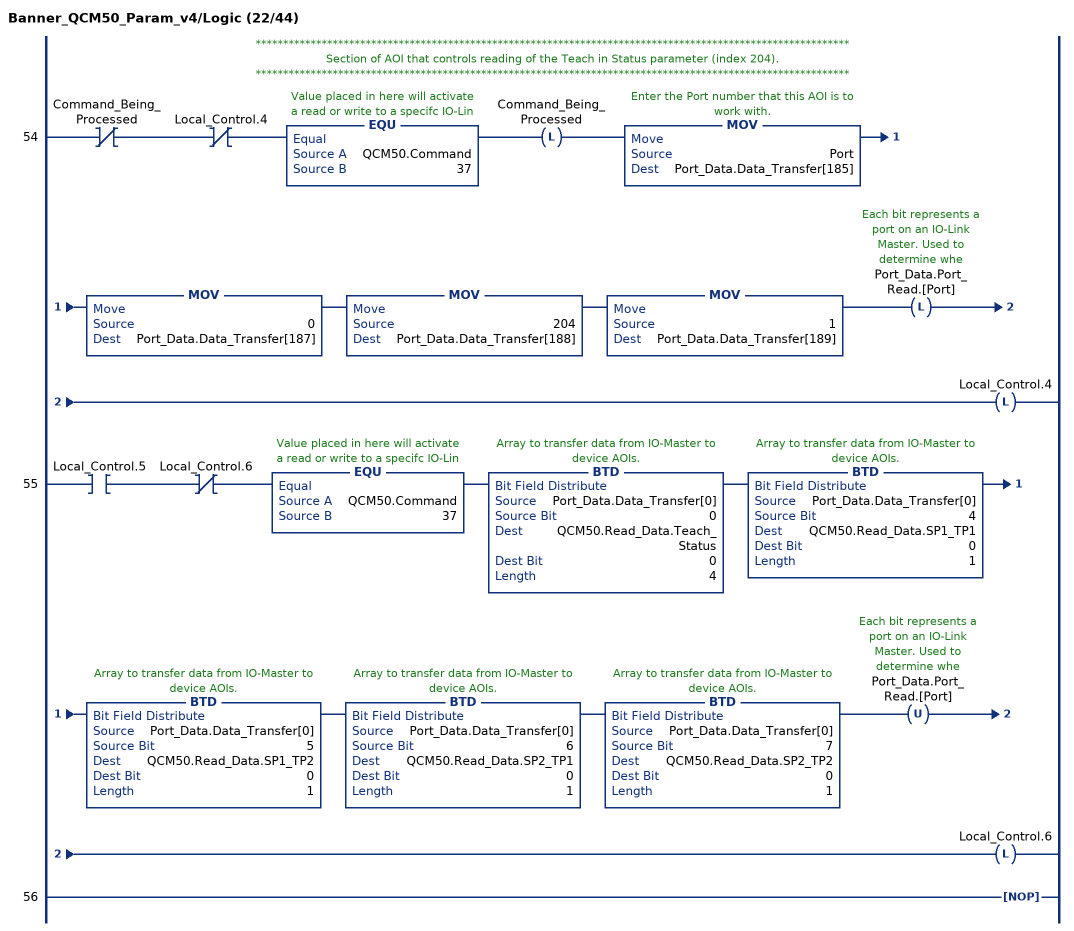
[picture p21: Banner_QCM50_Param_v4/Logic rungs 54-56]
   // ************************************************************************************************************
   // Section of AOI that controls reading of the Teach in Status parameter (index 204).
   // ************************************************************************************************************
   54: XIO(Command_Being_Processed)XIO(Local_Control.4)EQU(QCM50.Command,37)OTL(Command_Being_Processed)MOV(Port,Port_Data.Data_Transfer[185])MOV(0,Port_Data.Data_Transfer[187])MOV(204,Port_Data.Data_Transfer[188])MOV(1,Port_Data.Data_Transfer[189])OTL(Port_Data.Port_Read.[Port])OTL(Local_Control.4);
   55: XIC(Local_Control.5)XIO(Local_Control.6)EQU(QCM50.Command,37)BTD(Port_Data.Data_Transfer[0],0,QCM50.Read_Data.Teach_Status,0,4)BTD(Port_Data.Data_Transfer[0],4,QCM50.Read_Data.SP1_TP1,0,1)BTD(Port_Data.Data_Transfer[0],5,QCM50.Read_Data.SP1_TP2,0,1)BTD(Port_Data.Data_Transfer[0],6,QCM50.Read_Data.SP2_TP1,0,1)BTD(Port_Data.Data_Transfer[0],7,QCM50.Read_Data.SP2_TP2,0,1)OTU(Port_Data.Port_Read.[Port])OTL(Local_Control.6);
   56: NOP();
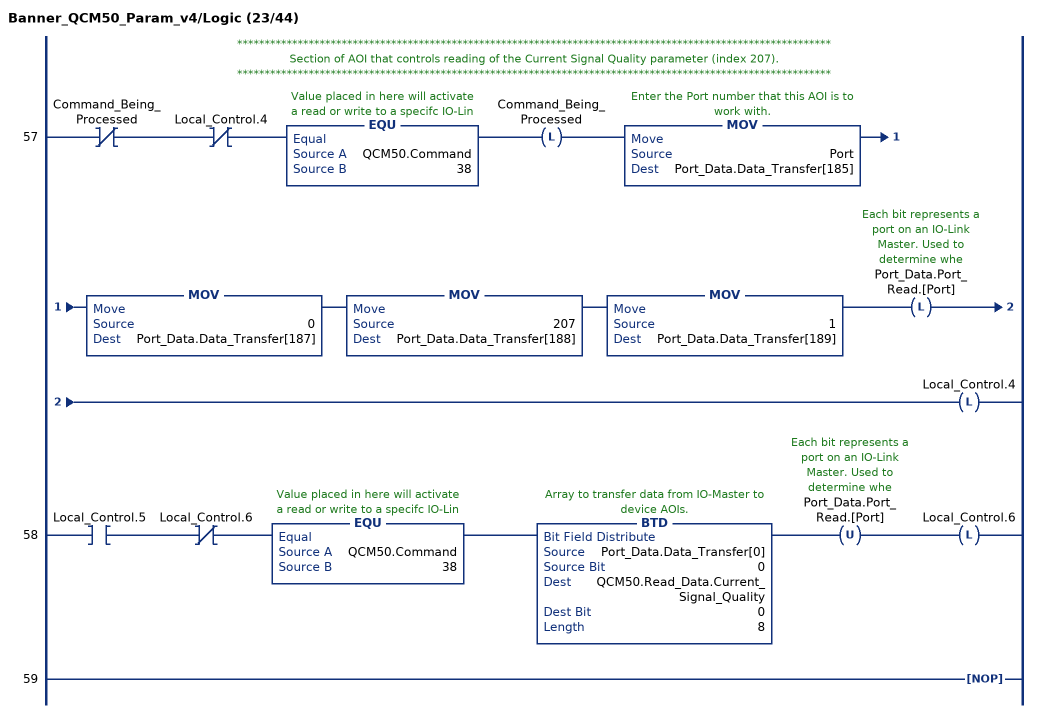
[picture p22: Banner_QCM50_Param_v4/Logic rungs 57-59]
   // ************************************************************************************************************
   // Section of AOI that controls reading of the Current Signal Quality parameter (index 207).
   // ************************************************************************************************************
   57: XIO(Command_Being_Processed)XIO(Local_Control.4)EQU(QCM50.Command,38)OTL(Command_Being_Processed)MOV(Port,Port_Data.Data_Transfer[185])MOV(0,Port_Data.Data_Transfer[187])MOV(207,Port_Data.Data_Transfer[188])MOV(1,Port_Data.Data_Transfer[189])OTL(Port_Data.Port_Read.[Port])OTL(Local_Control.4);
   58: XIC(Local_Control.5)XIO(Local_Control.6)EQU(QCM50.Command,38)BTD(Port_Data.Data_Transfer[0],0,QCM50.Read_Data.Current_Signal_Quality,0,8)OTU(Port_Data.Port_Read.[Port])OTL(Local_Control.6);
   59: NOP();
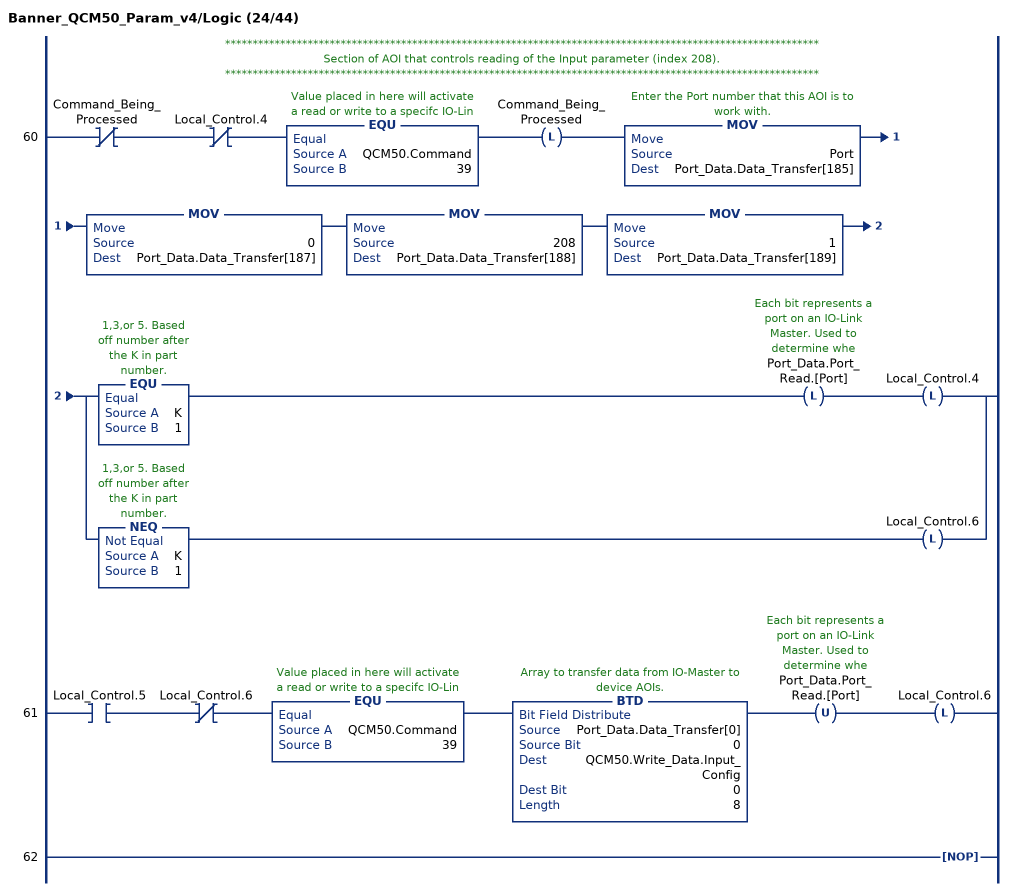
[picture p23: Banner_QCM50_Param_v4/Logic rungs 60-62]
   // ************************************************************************************************************
   // Section of AOI that controls reading of the Input parameter (index 208).
   // ************************************************************************************************************
   60: XIO(Command_Being_Processed)XIO(Local_Control.4)EQU(QCM50.Command,39)OTL(Command_Being_Processed)MOV(Port,Port_Data.Data_Transfer[185])MOV(0,Port_Data.Data_Transfer[187])MOV(208,Port_Data.Data_Transfer[188])MOV(1,Port_Data.Data_Transfer[189])[EQU(K,1) OTL(Port_Data.Port_Read.[Port]) OTL(Local_Control.4) ,NEQ(K,1) OTL(Local_Control.6) ];
   61: XIC(Local_Control.5)XIO(Local_Control.6)EQU(QCM50.Command,39)BTD(Port_Data.Data_Transfer[0],0,QCM50.Write_Data.Input_Config,0,8)OTU(Port_Data.Port_Read.[Port])OTL(Local_Control.6);
   62: NOP();
